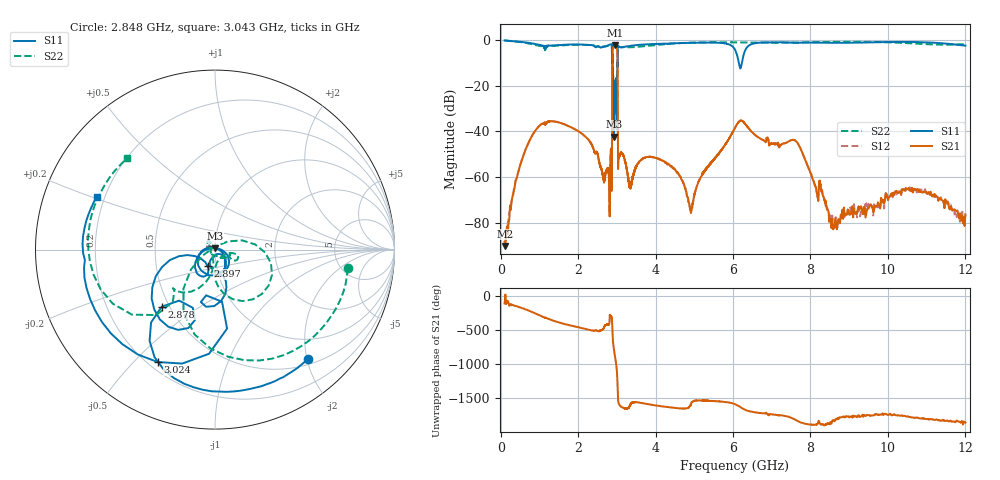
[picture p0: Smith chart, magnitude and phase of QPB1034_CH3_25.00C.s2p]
! TDS: k:\Engsetup\Winsaw\QPB1034_ALL
! Channel 1
! Ports=1 2
! seg 1=100.000000 1100.000000 51
! seg 2=1101.000000 1301.000000 201
! seg 3=1302.000000 2302.000000 101
! seg 4=2303.000000 3503.000000 1201
! seg 5=3504.000000 5204.000000 171
! seg 6=5205.000000 6405.000000 1201
! seg 7=6406.000000 8506.000000 211
! seg 8=8507.000000 12007.000000 176
! Points=3313
! FailCode=0
! Topology=ALL_SE(12)
!VNA Cal loaded =QPB1034_ALL_25C
!PS1(V)= 5.000
!PS(mA)= 0.427
!PS2(V)= 0.630
!PS(mA)= -0.002
!PS3(V)= 1.170
!PS(mA)= 0.000
!PS4(V)= 1.170
!PS(mA)= -0.001
!Temp (C)= 25.00
# MHz S DB R 50
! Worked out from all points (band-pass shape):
!   3313 points, 100 MHz to 12.01 GHz, reference 50 ohm
!   highest |S21| = -2.43 dB at 2.947 GHz (marker M1); lowest = -90.0 dB at 120 MHz (marker M2)
!   |S21| within 3 dB of the highest: 2.89 GHz to 3.014 GHz (123.4 MHz wide, 4.18 % of centre)
!   lowest |S11| = -42.3 dB at 2.919 GHz (marker M3), VSWR 1.02, Z = 49.9 + j0.765 ohm
!   |S11| at or under -10 dB: 2.89 GHz to 3.016 GHz (126.3 MHz wide, 4.28 % of centre); 3.017305 GHz to 3.020181 GHz (2.876 MHz wide, 0.0953 % of centre); 6.151 GHz to 6.231 GHz (80.25 MHz wide, 1.3 % of centre)
!   |S22| runs from -35.9 to -0.3 dB; largest |S21 - S12| = 0.005
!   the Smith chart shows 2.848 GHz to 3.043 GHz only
!   S11 on the Smith chart (normalised r, x): 2.848 GHz: 0.59, -2.01; 2.878 GHz: 0.45, -0.36; 2.897 GHz: 0.91, -0.17; 3.024 GHz: 0.24, -0.59; 3.043 GHz: 0.17, +0.21
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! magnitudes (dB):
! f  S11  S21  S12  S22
! 100 MHz  -0.3  -88.2  -90.1  -0.3
! 120 MHz  -0.3  -90.0  -87.4  -0.3
! 240 MHz  -0.5  -72.4  -74.7  -0.5
! 500 MHz  -0.9  -54.7  -54.9  -1.0
! 1.1 GHz  -2.5  -36.3  -36.4  -2.9
! 2.434 GHz  -3.0  -49.4  -49.2  -2.9
! 2.806 GHz  -2.2  -64.5  -64.7  -2.5
! 2.848 GHz  -1.9  -47.7  -47.7  -2.5
! 2.878 GHz  -7.2  -22.2  -22.2  -22.1
! 2.897 GHz  -20.0  -3.7  -3.7  -25.3
! 2.919 GHz  -42.3  -2.6  -2.7  -20.7
! 2.947 GHz  -20.8  -2.4  -2.4  -25.4
! 3.005 GHz  -18.1  -3.7  -3.7  -31.0
! 3.024 GHz  -3.1  -26.6  -26.6  -3.4
! 3.043 GHz  -2.8  -51.9  -51.9  -3.0
! 4.904 GHz  -1.3  -73.9  -73.6  -1.3
! 5.406 GHz  -1.2  -54.1  -54.2  -1.1
! 6.224 GHz  -10.6  -35.3  -35.3  -1.2
! 7.636 GHz  -1.3  -44.4  -44.4  -1.2
! 8.607 GHz  -1.3  -81.2  -82.6  -0.9
! 10.65 GHz  -1.0  -66.7  -65.2  -1.6
! 12.01 GHz  -2.5  -76.2  -76.3  -1.9
